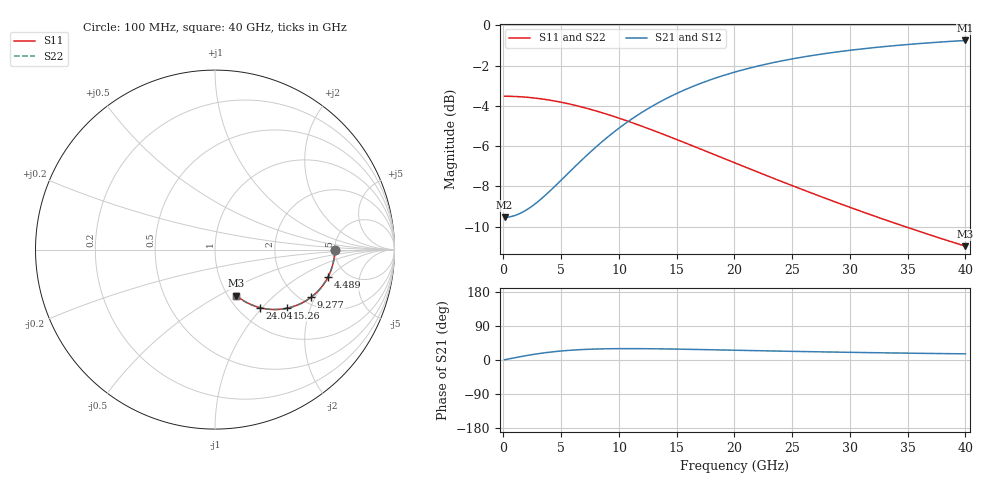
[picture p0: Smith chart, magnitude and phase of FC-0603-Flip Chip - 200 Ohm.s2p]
!Vishay Thin-Film
!FC Family
!Case Size 0603
!Assembly Style Flip Chip
!11/9/2015
!thinfilm@vishay.com
# GHz S MA R 50
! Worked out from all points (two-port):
!   101 points, 100 MHz to 40 GHz, reference 50 ohm
!   highest |S21| = -0.75 dB at 40 GHz (marker M1); lowest = -9.5 dB at 100 MHz (marker M2)
!   |S21| within 3 dB of the highest: 13.72 GHz to end of sweep
!   lowest |S11| = -11.0 dB at 40 GHz (marker M3), VSWR 1.79, Z = 54.7 - j30.5 ohm
!   |S11| at or under -10 dB: 34.78 GHz to end of sweep
!   |S22| runs from -11.0 to -3.5 dB; largest |S21 - S12| = 0
!   S11 on the Smith chart (normalised r, x): 100 MHz: 5.00, -0.06; 4.489 GHz: 3.64, -1.90; 9.277 GHz: 2.25, -1.85; 15.26 GHz: 1.57, -1.40; 24.04 GHz: 1.25, -0.97; 40 GHz: 1.09, -0.61
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0.1  0.6667 -0.3  0.3334 0.6  0.3334 0.6  0.6667 -0.3
0.898  0.6659 -2.7  0.3364 5.4  0.3364 5.4  0.6659 -2.7
2.095  0.6625 -6.4  0.3494 12.2  0.3494 12.2  0.6625 -6.4
3.292  0.6566 -10.0  0.3711 17.8  0.3711 17.8  0.6566 -10.0
4.489  0.6483 -13.5  0.3993 22.2  0.3993 22.2  0.6483 -13.5
5.686  0.638 -16.9  0.4314 25.4  0.4314 25.4  0.638 -16.9
6.883  0.6258 -20.2  0.4657 27.6  0.4657 27.6  0.6258 -20.2
8.08  0.6122 -23.3  0.5006 29.0  0.5006 29.0  0.6122 -23.3
9.277  0.5975 -26.4  0.5351 29.7  0.5351 29.7  0.5975 -26.4
11.272  0.5713 -31.1  0.5896 30.0  0.5896 30.0  0.5713 -31.1
12.469  0.5551 -33.7  0.6199 29.8  0.6199 29.8  0.5551 -33.7
13.666  0.5387 -36.1  0.6482 29.4  0.6482 29.4  0.5387 -36.1
15.262  0.517 -39.2  0.6827 28.6  0.6827 28.6  0.517 -39.2
17.656  0.4853 -43.3  0.7278 27.2  0.7278 27.2  0.4853 -43.3
20.05  0.4553 -47.0  0.7657 25.8  0.7657 25.8  0.4553 -47.0
22.045  0.4318 -49.7  0.7924 24.6  0.7924 24.6  0.4318 -49.7
24.04  0.4099 -52.1  0.8154 23.4  0.8154 23.4  0.4099 -52.1
26.833  0.3818 -55.2  0.8423 21.8  0.8423 21.8  0.3818 -55.2
30.025  0.353 -58.1  0.8671 20.2  0.8671 20.2  0.353 -58.1
33.616  0.3246 -61.0  0.889 18.6  0.889 18.6  0.3246 -61.0
36.808  0.3025 -63.1  0.9046 17.4  0.9046 17.4  0.3025 -63.1
40  0.2828 -65.0  0.9172 16.2  0.9172 16.2  0.2828 -65.0
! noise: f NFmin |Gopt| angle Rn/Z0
0.1  1.929e-15  1  -8.538e-07  3.999
4.489  0  1  -1.892e-15  2.636
8.878  1.211e-07  1  1.973e-14  1.323
13.27  9.643e-16  1  2.152e-14  0.724
17.66  4.056e-08  1  1.016e-14  0.4432
22.05  2.705e-08  1  -1.285e-14  0.2956
26.43  0  1  1.346e-14  0.2099
30.82  0  1  1.004e-14  0.1561
35.21  0  1  3.487e-14  0.1204
40  1.212e-08  1  2.524e-15  0.09361
